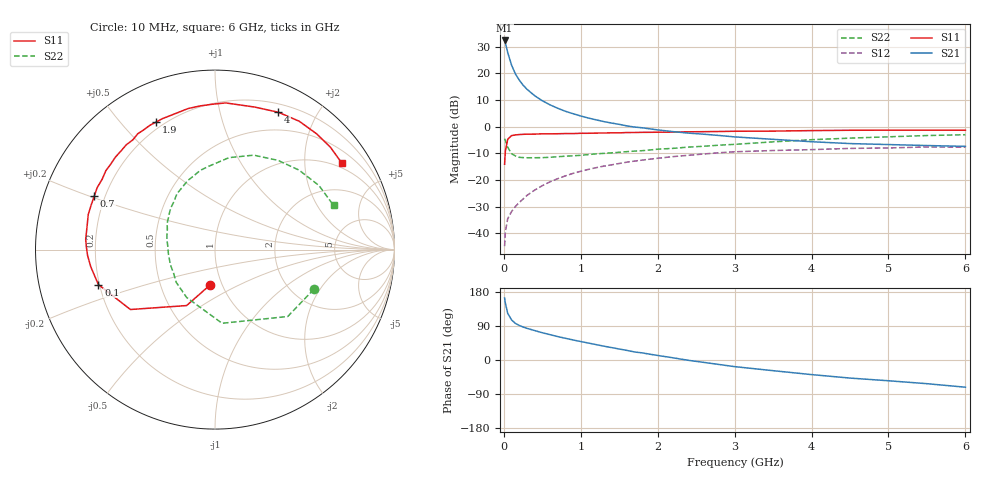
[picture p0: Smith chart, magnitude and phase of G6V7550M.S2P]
! SIEMENS Small Signal Semiconductors
! BFG193
! Si NPN RF Bipolar Junction Transistor in SOT223
! VCE = 0.75 V  IC = 50 mA
! Common Emitter S-Parameters:  August  1996
# GHz  S  MA  R  50
!  f  S11  S21  S12  S22
! GHz  MAG  ANG  MAG  ANG  MAG  ANG  MAG  ANG
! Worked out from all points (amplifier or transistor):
!   36 points, 10 MHz to 6 GHz, reference 50 ohm
!   highest |S21| = 32.4 dB at 10 MHz (marker M1)
!   |S21| within 3 dB of that: start of sweep to 37.53 MHz
!   unconditionally stable (mu >= 1): start of sweep to 14.82 MHz; 173.1 MHz to end of sweep
!   at 250 MHz: K = 1.11, MAG = 19.4 dB, |S12| = -27.2 dB
!   at 1.4 GHz: K = 1.18, MAG = 5.3 dB, |S12| = -14.3 dB
!   at 6 GHz: K = 1.07, MAG = -1.4 dB, |S12| = -7.7 dB
!   S11 on the Smith chart (normalised r, x): 10 MHz: 0.88, -0.36; 100 MHz: 0.20, -0.14; 700 MHz: 0.16, +0.21; 1.9 GHz: 0.17, +0.63; 4 GHz: 0.29, +1.53; 6 GHz: 0.84, +3.03
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0.01  0.197 -97.4  41.52 163.4  0.0057 73.0  0.5933 -21.9
0.02  0.3497 -116.9  37.43 149.9  0.0106 64.1  0.5506 -42.6
0.05  0.5776 -144.7  24.74 123.3  0.0187 52.2  0.4124 -84.5
0.1  0.6783 -163.3  14.34 105.8  0.0254 51.9  0.31 -120.7
0.15  0.699 -172.2  9.816 96.6  0.0317 54.8  0.2825 -140.0
0.2  0.7108 -177.4  7.506 91.3  0.0375 57.8  0.2653 -150.6
0.25  0.7172 178.6  6.017 87.0  0.0438 59.9  0.2624 -159.6
0.3  0.7228 175.4  5.043 83.6  0.0511 61.3  0.2605 -164.9
0.4  0.7243 169.8  3.816 77.7  0.0642 62.0  0.2608 -174.5
0.5  0.7328 164.5  3.065 71.9  0.078 61.5  0.2617 178.8
0.6  0.7333 160.3  2.568 66.9  0.092 60.7  0.2661 173.6
0.7  0.7358 156.1  2.215 61.8  0.1054 59.1  0.2724 168.9
0.9  0.7409 148.1  1.749 52.9  0.1328 55.0  0.2834 159.8
1.1  0.7511 140.7  1.448 44.7  0.1574 50.7  0.299 152.9
1.5  0.7638 126.8  1.104 29.0  0.2033 40.7  0.3302 139.6
1.9  0.7827 114.8  0.909 15.2  0.2454 30.9  0.3647 127.1
2.2  0.7891 106.4  0.806 5.8  0.2737 22.9  0.3913 118.0
3.5  0.8244 74.4  0.578 -28.2  0.3565 -10.3  0.5181 81.4
4  0.8428 65.2  0.521 -38.5  0.3701 -19.9  0.5688 67.7
4.5  0.8554 56.7  0.481 -47.7  0.3902 -29.5  0.6086 54.8
5.5  0.8597 41.7  0.442 -62.5  0.4158 -51.3  0.6805 31.6
6  0.8554 34.3  0.426 -71.8  0.4117 -63.6  0.7049 20.5
